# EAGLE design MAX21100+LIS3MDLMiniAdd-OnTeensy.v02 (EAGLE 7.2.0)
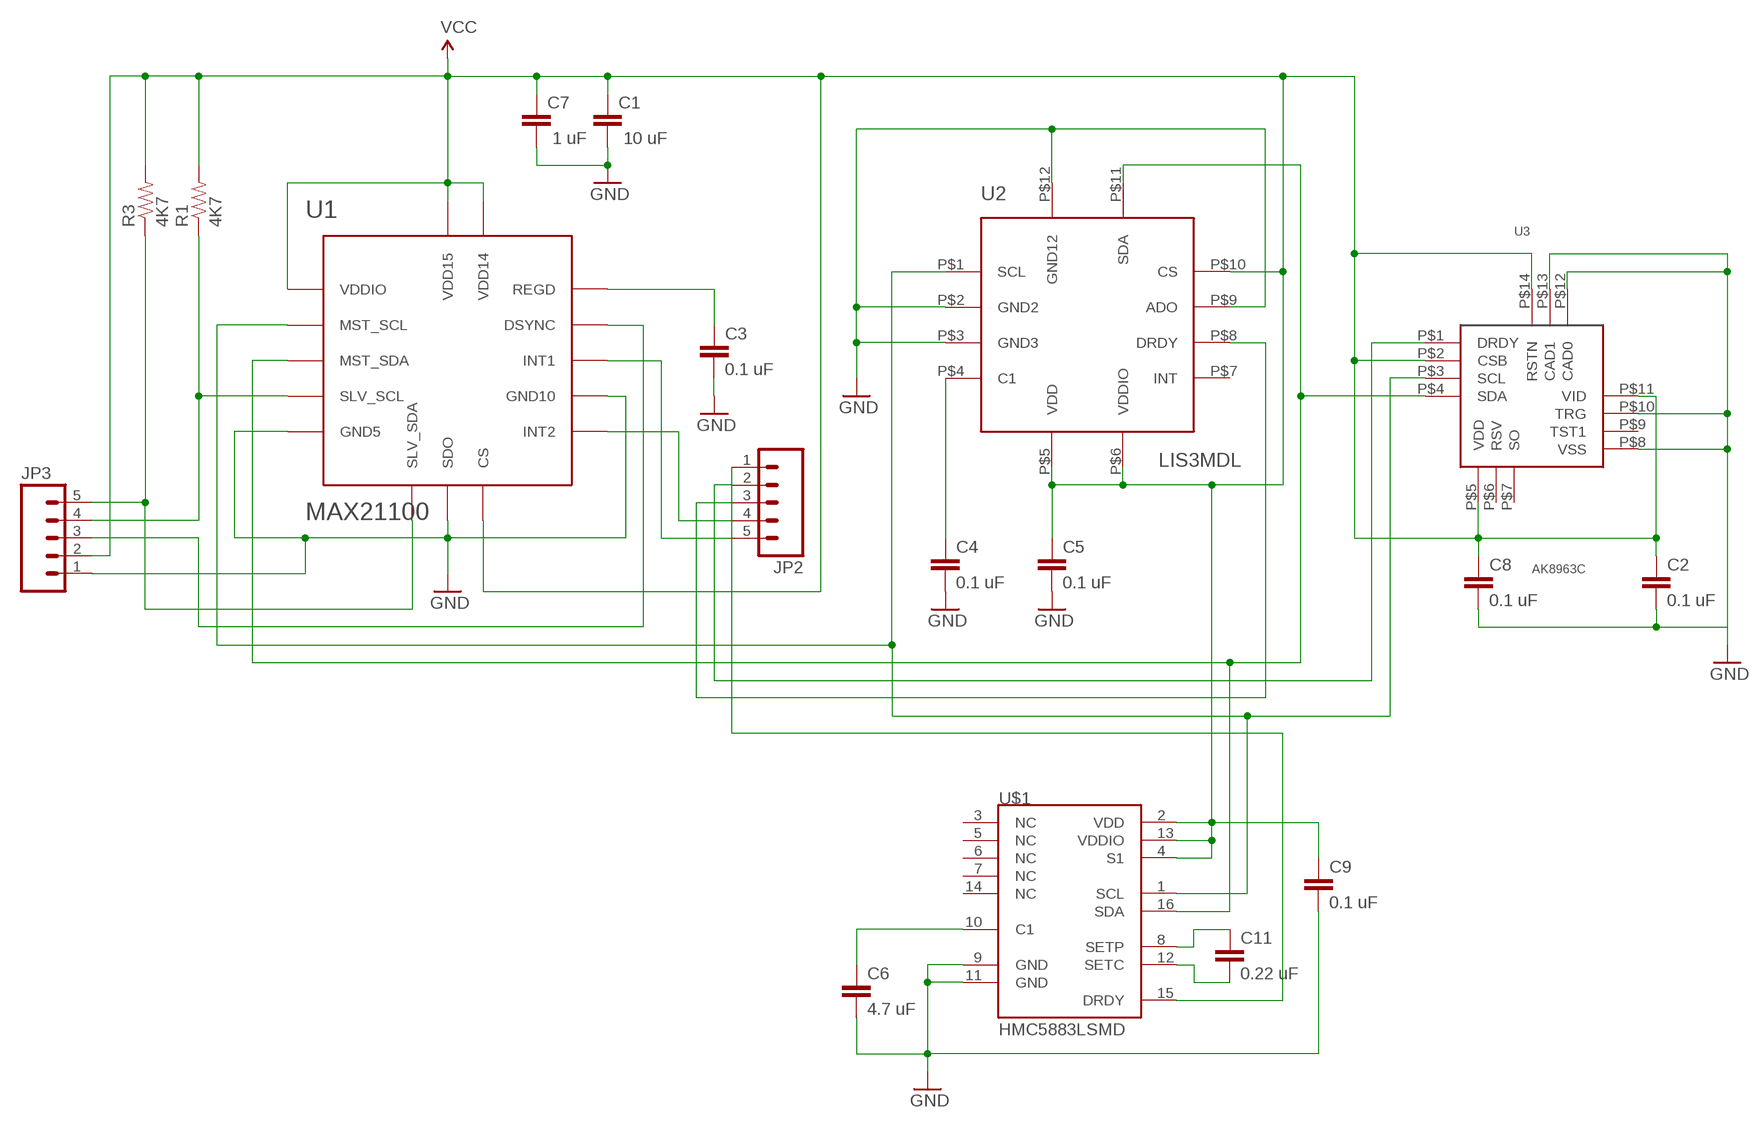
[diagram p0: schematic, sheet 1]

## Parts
C1  10 uF  0402CAP.KW  [0402-CAP]
C2  0.1 uF  0402CAP.KW  [0402-CAP]
C3  0.1 uF  0402CAP.KW  [0402-CAP]
C4  0.1 uF  0402CAP.KW  [0402-CAP]
C5  0.1 uF  0402CAP.KW  [0402-CAP]
C6  4.7 uF  0402CAP.KW  [0402-CAP]
C7  1 uF  0402CAP.KW  [0402-CAP]
C8  0.1 uF  0402CAP.KW  [0402-CAP]
C9  0.1 uF  0402CAP.KW  [0402-CAP]
C11  0.22 uF  0402CAP.KW  [0402-CAP]
JP2  M05NO_SILK  [1X05_NO_SILK]
JP3  M05NO_SILK  [1X05_NO_SILK]
R1  4K7  0402RES.KW  [0402-RES]
R3  4K7  0402RES.KW  [0402-RES]
U1  MAX21100  [LGA-16]
U2  LIS3MDL  [VFLGA-12]
U3  AK8963C  [AK8963C]
U$1  HMC5883LSMD  [16LPCC]

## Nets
GND: C1.2 C2.2 C3.2 C4.2 C5.2 C6.2 C7.2 C8.2 C9.2 JP3.1 U1.P$5(GND5) U1.P$7(SDO) U1.P$10(GND10) U2.P$2(GND2) U2.P$3(GND3) U2.P$9(ADO) U2.P$12(GND12) U3.P$8(VSS) U3.P$10(TRG) U3.P$12(CAD0) U3.P$13(CAD1) U$1.9(GND) U$1.11(GND)
N$1: JP2.3 U2.P$8(DRDY)
N$2: JP2.2 U3.P$1(DRDY)
N$3: C3.1 U1.P$13(REGD)
N$4: C6.1 U$1.10(C1)
N$6: JP3.4 R1.1 U1.P$4(SLV_SCL)
N$7: JP3.5 R3.1 U1.P$6(SLV_SDA)
N$9: JP2.1 U$1.15(DRDY)
N$10: JP2.5 U1.P$11(INT1)
N$11: JP2.4 U1.P$9(INT2)
N$12: JP3.3 U1.P$12(DSYNC)
N$13: U1.P$2(MST_SCL) U2.P$1(SCL) U3.P$3(SCL) U$1.1(SCL)
N$14: U1.P$3(MST_SDA) U2.P$11(SDA) U3.P$4(SDA) U$1.16(SDA)
N$15: C4.1 U2.P$4(C1)
N$17: C11.1 U$1.8(SETP)
N$18: C11.2 U$1.12(SETC)
VCC: C1.1 C2.1 C5.1 C7.1 C8.1 C9.1 JP3.2 R1.2 R3.2 U1.P$1(VDDIO) U1.P$8(CS) U1.P$14(VDD14) U1.P$15(VDD15) U2.P$5(VDD) U2.P$6(VDDIO) U2.P$10(CS) U3.P$2(CSB) U3.P$5(VDD) U3.P$11(VID) U3.P$14(RSTN) U$1.2(VDD) U$1.4(S1) U$1.13(VDDIO)
Unconnected: U2.P$7(INT) U3.P$6(RSV) U3.P$7(SO) U3.P$9(TST1) U$1.3(NC) U$1.5(NC) U$1.6(NC) U$1.7(NC) U$1.14(NC)

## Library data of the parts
C1-C9 C11 = SparkFun-Capacitors:0402CAP.KW
JP2 JP3 = SparkFun-Connectors:M05: Header 5 Standard 5-pin 0.1" header. Use with straight break away headers (SKU : PRT-00116), right angle break away headers (PRT-00553), swiss pins (PRT-00743), machine pins (PRT-00117), and female headers (PRT-00115). Molex polarized connector foot print use with SKU : PRT-08230 with associated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
R1 R3 = SparkFun-Resistors:0402RES.KW
U1 = SparkFun-DigitalIC:MAX21100: MAX2110 6 + 3 DoF motion sensor in LGA-16 package
U2 = SparkFun-DigitalIC:LIS3MDL: LIS3MDL magnetometer in a VFLGA-12 package
U3 = Kris:AK8963C: BGA-14 package for AK8963C magnetometer
U$1 = SparkFun-Sensors:HMC5883L: 3 Axis Digital Compass IC

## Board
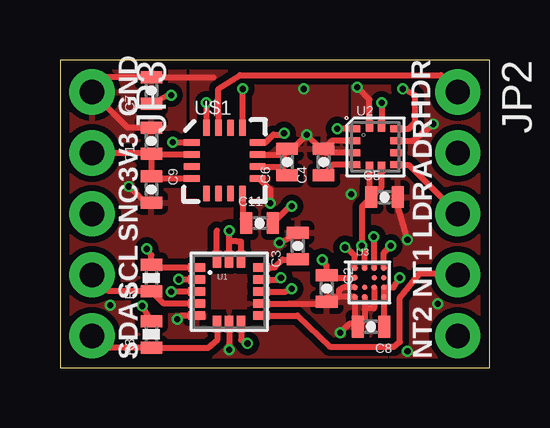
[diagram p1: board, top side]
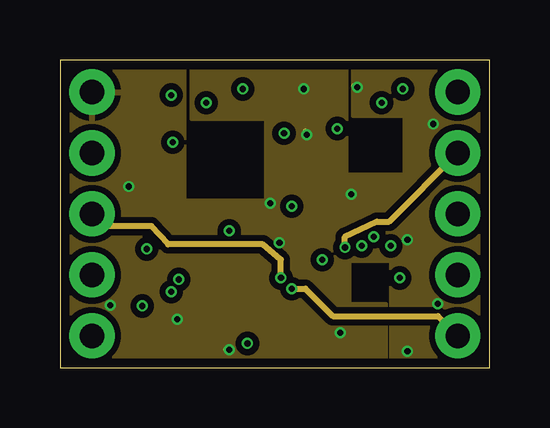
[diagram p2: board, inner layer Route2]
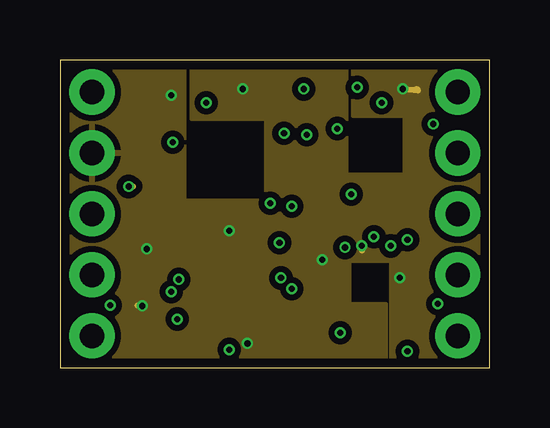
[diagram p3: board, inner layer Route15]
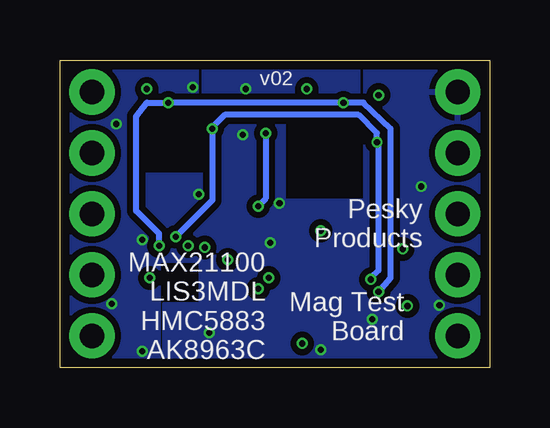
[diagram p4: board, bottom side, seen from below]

Size 17.91 x 12.83 mm. Coordinates in mm from the lower left corner, seen from the top.
Outline: 0,0 17.91,0 17.91,12.83 0,12.83 0,0
Copper layers (1*2*15*16): Top 0.035559375mm / dielectric 0.17018125mm / Route2 0.01778125mm / dielectric 47mil / Route15 0.01778125mm / dielectric 0.17018125mm / Bottom 0.035559375mm
Design rules "OSHPark-4layer *": minimum track width 5mil, minimum drill 10mil, track to track 5mil, track to pad 5mil, pad to pad 5mil, via to via 5mil, smd to smd 5mil, copper to edge 15mil, drill to drill 6mil, minimum pad ring 4mil, minimum via ring 4mil, stop-mask expansion 4mil, vias tented up to drill 20mil, thermal gap 10mil

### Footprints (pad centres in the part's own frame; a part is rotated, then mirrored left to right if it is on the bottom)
0402-CAP = smd 0.5 x 0.9: 1 -0.55,0; 2 0.55,0
1X05_NO_SILK = drill 1.016 pad 1.88: 1 0,0; 2 2.54,0; 3 5.08,0; 4 7.62,0; 5 10.16,0
0402-RES = smd 0.5 x 0.9: 1 -0.55,0; 2 0.55,0
LGA-16 = smd 0.7 x 0.35: P$1 -1.35,1; P$2 -1.35,0.5; P$3 -1.35,0; P$4 -1.35,-0.5; P$5 -1.35,-1; P$9 1.35,-1; P$10 1.35,-0.5; P$11 1.35,0; P$12 1.35,0.5; P$13 1.35,1 | smd 0.35 x 0.7: P$6 -0.5,-1.35; P$7 0,-1.35; P$8 0.5,-1.35; P$14 0.5,1.35; P$15 0,1.35; P$16 -0.5,1.35
VFLGA-12 = smd 0.475 x 0.3: P$1 -0.863,0.75; P$2 -0.863,0.25; P$3 -0.863,-0.25; P$4 -0.863,-0.75; P$7 0.863,-0.25; P$8 0.863,-0.75; P$9 0.863,0.25; P$10 0.863,0.75 | smd 0.3 x 0.475: P$5 -0.25,-0.863; P$6 0.25,-0.863; P$11 0.25,0.863; P$12 -0.25,0.863
AK8963C = smd 0.23 x 0.23: P$1 -0.6,0.6; P$2 -0.2,0.6; P$3 0.2,0.6; P$4 0.6,0.6; P$5 -0.6,0.2; P$6 0.2,0.2; P$7 0.6,0.2; P$8 -0.6,-0.2; P$9 -0.2,-0.2; P$10 0.2,-0.2; P$11 0.6,-0.2; P$12 -0.6,-0.6; P$13 -0.2,-0.6; P$14 0.6,-0.6
16LPCC = smd 0.65 x 0.28: 1 -1.37,0.75; 2 -1.37,0.25; 3 -1.37,-0.25; 4 -1.37,-0.75; 9 1.37,-0.75; 10 1.37,-0.25; 11 1.37,0.25; 12 1.37,0.75 | smd 0.28 x 0.65: 5 -0.75,-1.37; 6 -0.25,-1.37; 7 0.25,-1.37; 8 0.75,-1.37; 13 0.75,1.37; 14 0.25,1.37; 15 -0.25,1.37; 16 -0.75,1.37

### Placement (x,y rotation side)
C1  3.81,9.46 90 top
C2  11.11,3.3 270 top
C3  9.91,5.08 90 top
C4  10.99,8.57 90 top
C5  13.53,7.11 0 top
C6  9.46,8.57 90 top
C7  3.81,11.56 90 top
C8  12.95,1.71 180 top
C9  3.81,7.43 270 top
C11  8.32,6.03 0 top
JP2  16.57,11.49 270 top
JP3  1.33,11.49 270 top
R1  3.81,3.75 90 top
R3  3.81,1.4 90 top
U1  7.05,3.17 0 top
U2  13.14,9.21 0 top
U3  12.89,3.56 0 top
U$1  6.86,8.64 0 top

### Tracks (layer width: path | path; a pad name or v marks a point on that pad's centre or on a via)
GND  (via drill 0.25)
  Top 0.254: 6.39,12.11 C7.2 1.82,12.11 JP3.1 2.82,10.01 C1.2 | U$1.11 9.35,8.89 9.35,9.01 C6.2 9.69,9.12 v10.29,9.72 10.88,9.12 C4.2 | U2.P$3 11.09,8.96 C4.2 | C9.2 3.6,6.88 v2.86,7.56 | U1.P$5 5.03,2.17 v4.89,2.03 | 11.62,2.96 U3.P$12 12.29,1.83 | 11.62,2.96 11.16,2.96 C2.2 11.04,2.67 U1.P$10 | U$1.9 8.31,7.89 8.76,7.43 v8.76,6.86 | U2.P$2 11.32,9.46 C4.2 | U1.P$7 v7.05,0.76 | C3.2 10.01,5.63 v9.14,5.21 | 12.29,1.83 12.05,1.83 v11.68,1.46 | 12.29,1.83 C8.2 12.69,2 12.69,2.41 | U2.P$12 12.89,11.17 v12.38,11.68 | U2.P$9 14.73,9.46 v15.56,10.16 | C5.2 14.07,6.69 v14.48,5.33 | U3.P$8 11.82,3.36 11.62,3.24 11.62,2.96 | U3.P$13 12.69,2.41 | U3.P$10 13.09,2.53 13.08,2.48 12.75,2.48 12.69,2.41
  Route2 0.254: v4.89,2.03 4.83,1.97 | 8.83,6.79 v8.76,6.86 8.7,6.92 | v10.29,9.72 10.29,9.78 10.22,9.84 | v7.05,0.76 6.92,0.76 | v11.68,1.46 11.56,1.46 | v12.38,11.68 12.32,11.68 12.26,11.75
  Route15 0.254: v2.86,7.56 3.05,7.56
  other vias: 10.16,11.62 15.75,2.67 2.1,2.6 12.13,7.24 14.48,0.7
  pour Route2 (isolate 0.254): 0,12.83 5.21,12.83 5.21,6.99 8.57,6.99 8.57,10.35 5.46,10.35 5.46,12.83 11.94,12.83 11.94,8.06 14.35,8.06 14.35,10.48 12.19,10.48 12.19,12.83 17.91,12.83 17.91,0 13.78,0 13.78,4.45 12.06,4.45 12.06,2.67 13.59,2.67 13.59,0 0,0
  pour Bottom (isolate 0.254): 0,12.83 5.21,12.83 5.21,6.99 8.57,6.99 8.57,10.35 5.46,10.35 5.46,12.83 11.94,12.83 11.94,8.06 14.35,8.06 14.35,10.48 12.19,10.48 12.19,12.83 17.91,12.83 17.91,0 13.78,0 13.78,4.45 12.06,4.45 12.06,2.67 13.59,2.67 13.59,0 0,0
  pour Top (isolate 0.254): 0,12.83 5.21,12.83 5.21,6.99 8.57,6.99 8.57,10.35 5.46,10.35 5.46,12.83 11.94,12.83 11.94,8.06 14.35,8.06 14.35,10.48 12.19,10.48 12.19,12.83 17.91,12.83 17.91,0 13.78,0 13.78,4.45 12.06,4.45 12.06,2.67 13.59,2.67 13.59,0 0,0
N$1
  Top 0.254: U2.P$8 14.53,8.46 JP2.3
N$2  (via drill 0.25)
  Top 0.254: U3.P$1 12.29,4.66 12.06,4.89 v11.87,5.02
  Route2 0.254: v11.87,5.02 11.87,5.46 13.21,6.1 13.72,6.1 JP2.2
N$3
  Top 0.254: U1.P$13 8.81,4.17 8.83,4.19 8.95,4.19 9.27,4.51 9.88,4.51 C3.1
N$4
  Top 0.254: U$1.10 9.22,8.39 C6.1
N$5
  Top 0.254: 6.54,4.51 6.54,5.71
N$6
  Top 0.254: U1.P$4 4.33,2.67 R1.1 2.01,3.2 JP3.4
N$7
  Top 0.254: JP3.5 1.82,0.85 R3.1 3.83,0.83 6.16,0.83 6.55,1.15 U1.P$6
N$9
  Top 0.254: U$1.15 6.61,10.6 6.6,10.6 6.6,11.62 7.49,12.19 15.88,12.19 JP2.1
N$10  (via drill 0.25)
  Top 0.254: U1.P$11 9.4,3.17 v9.65,3.3
  Route2 0.254: v9.65,3.3 10.22,3.3 11.37,2.16 15.75,2.16 JP2.5
N$11
  Top 0.254: U1.P$9 9.89,2.17 11.24,0.89 13.91,0.89 14.16,1.08 14.16,2.92 14.99,3.94 16.51,3.94 JP2.4
N$12  (via drill 0.25)
  Top 0.254: U1.P$12 9.14,3.67 v9.21,3.75
  Route2 0.254: v9.21,3.75 9.21,4.51 8.45,5.14 4.51,5.14 3.81,5.91 1.84,5.91 JP3.3
N$13  (via drill 0.25)
  Top 0.254: U1.P$2 4.96,3.67 v4.95,3.68 | 5.48,9.4 U$1.1 4.71,9.39 v4.7,9.4 | v13.08,5.46 U3.P$3 | U2.P$1 11.67,9.96 v11.56,9.97
  Bottom 0.254: v4.95,3.68 4.95,3.75 4.64,4.06 4.64,9.21 v4.7,9.4 4.7,9.78 5.46,10.54 11.05,10.54 11.56,10.03 v11.56,9.97 11.56,6.99 v13.08,5.46
N$14  (via drill 0.25)
  Top 0.254: U1.P$3 v4.64,3.17 | v13.4,11.05 U2.P$11 | v6.1,11.05 6.1,10.02 U$1.16 | U3.P$4 13.49,4.79 v13.78,5.08
  Bottom 0.254: v4.64,3.17 4.13,3.75 4.13,9.97 5.27,11.05 v6.1,11.05 v13.4,11.05 14.29,11.05 14.73,10.48 14.73,6.54 13.78,5.59 v13.78,5.08
N$15
  Top 0.254: U2.P$4 11.36,8.46 C4.1
N$17
  Top 0.254: U$1.8 7.61,6.19 C11.1
N$18  (via drill 0.25)
  Top 0.254: U$1.12 8.56,9.39 8.89,9.72 9.21,9.72 v9.34,9.78 | v9.65,6.73 9.57,6.73 C11.2
  Bottom 0.254: v9.34,9.78 9.34,7.05 v9.65,6.73
VCC  (via drill 0.25)
  Top 0.254: JP3.2 3.77,8.95 C1.1 | U$1.2 3.84,8.89 C1.1 | C1.1 C9.1 3.9,7.89 U$1.4 | C7.1 4.53,11.39 v4.64,11.37 | U1.P$1 3.93,4.17 R1.2 3.81,4.7 v3.62,4.95 | R3.2 3.81,1.97 v3.43,2.58 | C8.1 13.49,1.73 U3.P$14 U3.P$11 13.9,3.36 v14.16,3.75 | U3.P$2 12.69,4.94 v12.57,5.08 12.57,6.71 C5.1 | U2.P$5 12.89,7.19 C5.1 | U2.P$6 13.39,7.53 C5.1 | U1.P$8 7.55,1.15 v7.81,1.02 | U1.P$14 7.55,5.26 7.37,5.27 7.05,5.27 | v10.92,4.51 11.11,4.25 C2.1 11.21,3.76 U3.P$5 | U2.P$10 14.53,9.96 14.8,10.22 14.8,11.37 v14.29,11.62 | U$1.13 7.61,11.61 v7.62,11.62 | U1.P$15 7.05,5.27 | 7.05,5.27 v7.05,5.71
  Route15 0.254: v3.62,4.95 3.68,5.02 | v3.43,2.58 3.24,2.6 | v12.57,5.08 12.57,4.89 | v14.16,3.75 14.16,3.81 | v10.92,4.51 10.86,4.51 | v14.29,11.62 14.92,11.56 14.86,11.62 | v7.62,11.62 7.68,11.68
  pour Route15 (isolate 0.254): 0,12.83 5.21,12.83 5.21,6.99 8.57,6.99 8.57,10.35 5.46,10.35 5.46,12.83 11.94,12.83 11.94,8.06 14.35,8.06 14.35,10.48 12.19,10.48 12.19,12.83 17.91,12.83 17.91,0 13.78,0 13.78,4.45 12.06,4.45 12.06,2.67 13.59,2.67 13.59,0 0,0

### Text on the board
tPlace: GND | HDR | 3V3 | ADR | SNC | LDR | SCL | NT1 | SDA | NT2
bPlace: v02 | Pesky / Products | MAX21100 / LIS3MDL / HMC5883 / AK8963C | Mag Test / Board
